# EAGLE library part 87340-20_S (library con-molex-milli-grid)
RECEPTACAL
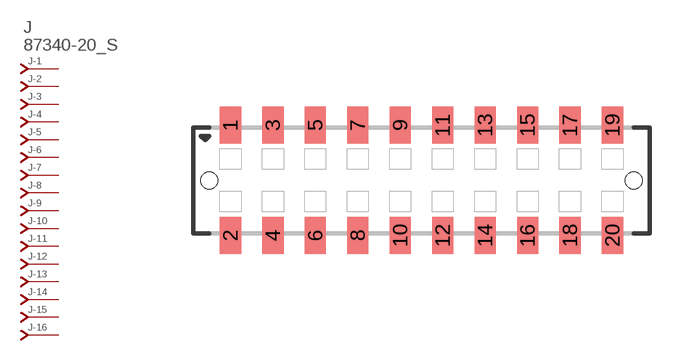
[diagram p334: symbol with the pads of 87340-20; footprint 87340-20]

Designator prefix J; gates -1=J-NV -2=J-N -3=J-N -4=J-N -5=J-N -6=J-N -7=J-N -8=J-N -9=J-N -10=J-N -11=J-N -12=J-N -13=J-N -14=J-N -15=J-N -16=J-N -17=J-N -18=J-N -19=J-N -20=J-N

## 87340-20_S  [87340-20]
1  -1:J  pas
2  -2:J  pas
3  -3:J  pas
4  -4:J  pas
5  -5:J  pas
6  -6:J  pas
7  -7:J  pas
8  -8:J  pas
9  -9:J  pas
10  -10:J  pas
11  -11:J  pas
12  -12:J  pas
13  -13:J  pas
14  -14:J  pas
15  -15:J  pas
16  -16:J  pas
17  -17:J  pas
18  -18:J  pas
19  -19:J  pas
20  -20:J  pas

## Footprint 87340-20 (pad centres in mm)
RECEPTACAL SMD Dual Row, Vertical, Low Profile
smd 1 x 1.75: 1 -9,2.6; 2 -9,-2.6; 3 -7,2.6; 4 -7,-2.6; 5 -5,2.6; 6 -5,-2.6; 7 -3,2.6; 8 -3,-2.6; 9 -1,2.6; 10 -1,-2.6; 11 1,2.6; 12 1,-2.6; 13 3,2.6; 14 3,-2.6; 15 5,2.6; 16 5,-2.6; 17 7,2.6; 18 7,-2.6; 19 9,2.6; 20 9,-2.6
hole 0.8 at -10,0
hole 0.8 at 10,0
